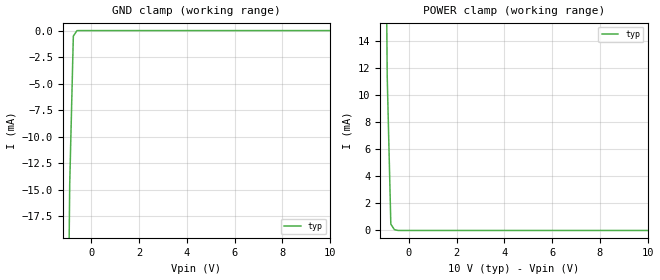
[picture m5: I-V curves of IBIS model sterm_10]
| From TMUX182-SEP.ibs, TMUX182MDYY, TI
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| sterm_10
[Model]   sterm_10
Model_type   Terminator
|   typ   min   max
C_comp   4.014581e-12   NA   NA
[Voltage Range]   10   NA   NA
[Temperature Range]   27   NA   NA
[Power Clamp Reference]   10   NA   NA
[GND Clamp Reference]   0   NA   NA
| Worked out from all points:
|   GND clamp passes 1 mA (typ) near -0.76 V on its own axis
|   POWER clamp passes 1 mA (typ) near -0.76 V on its own axis
[GND Clamp]
|   Voltage   I(typ)   I(min)   I(max)
-5V       -2.321A    NA         NA
-1.061V   -47.66mA   NA         NA
-909.1mV  -14.48mA   NA         NA
-757.6mV  -521uA     NA         NA
-606.1mV  -5.734uA   NA         NA
10V       106.8pA    NA         NA
[POWER Clamp]
|   Voltage   I(typ)   I(min)   I(max)
-5V       1.914A     NA         NA
-1.061V   43.19mA    NA         NA
-909.1mV  11.39mA    NA         NA
-757.6mV  467.9uA    NA         NA
-606.1mV  57.27uA    NA         NA
-303mV    750.9pA    NA         NA
10V       -58.07pA   NA         NA
